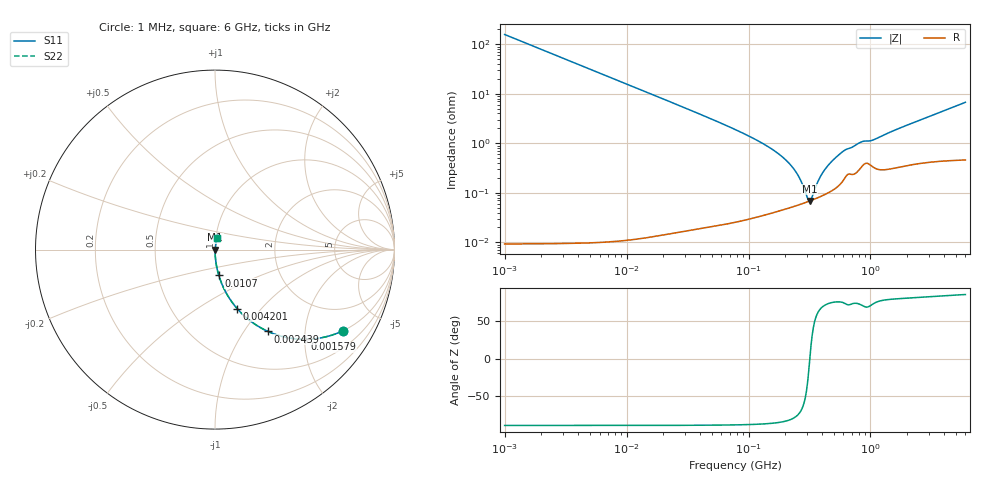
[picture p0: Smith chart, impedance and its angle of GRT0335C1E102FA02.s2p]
!Murata Part Number: GRT0335C1E102FA02
!These Parameters are Measured in Series Mode Connection
!Data Generated on Jun 19, 2026
!  o--ll--o
!Port1  Port2
!  o------o
!Operation Temp=25[degC], DC Bias Voltage=0[V]
!Freq. Start=1000[kHz] Stop=6[GHz] 401[Steps]
# Hz S RI R 50
!Freq.(Hz) S11(Real) S11(Imag) S21(Real) S21(Imag) S12(Real) S12(Imag) S22(Real) S22(Imag)
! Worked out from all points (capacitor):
!   401 points, 1 MHz to 6 GHz, reference 50 ohm
!   read as one part in series: C = 1.01 nF near 1.044 MHz
!   lowest |Z| = 68.5 mohm at 318.4 MHz (marker M1)
!   series resonance near 318.1 MHz, so ESL is about 250 pH
!   S11 on the Smith chart (normalised r, x): 1 MHz: 1.00, -3.15; 1.579 MHz: 1.00, -2.00; 2.439 MHz: 1.00, -1.29; 4.201 MHz: 1.00, -0.75; 10.7 MHz: 1.00, -0.29; 6 GHz: 1.01, +0.13
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1000000  0.7133 -0.4522  0.2867 0.4522  0.2867 0.4522  0.7133 -0.4522
1578894  0.4995 -0.5  0.5005 0.5  0.5005 0.5  0.4995 -0.5
2439274  0.2948 -0.4559  0.7052 0.4559  0.7052 0.4559  0.2948 -0.4559
4201409  0.1235 -0.3289  0.8765 0.3289  0.8765 0.3289  0.1235 -0.3289
4293785  0.1189 -0.3235  0.8811 0.3235  0.8811 0.3235  0.1189 -0.3235
1.0704e7  0.0213 -0.144  0.9787 0.144  0.9787 0.144  0.0213 -0.144
1.843659e7  0.00734 -0.0846  0.9927 0.0846  0.9927 0.0846  0.00734 -0.0846
7.745967e7  0.000615 -0.019  0.9994 0.019  0.9994 0.019  0.000615 -0.019
1.39348e8  0.000443 -0.00904  0.9996 0.00904  0.9996 0.00904  0.000443 -0.00904
2.016844e8  0.000491 -0.0046  0.9995 0.0046  0.9995 0.0046  0.000491 -0.0046
2.506837e8  0.000562 -0.00234  0.9994 0.00234  0.9994 0.00234  0.000562 -0.00234
2.734687e8  0.0006 -0.00148  0.9994 0.00148  0.9994 0.00148  0.0006 -0.00148
3.048839e8  0.000658 -0.000413  0.9993 0.000413  0.9993 0.000413  0.000658 -0.000413
3.184382e8  0.000685 1e-05  0.9993 -1e-05  0.9993 -1e-05  0.000685 1e-05
3.325952e8  0.000714 0.000433  0.9993 -0.000433  0.9993 -0.000433  0.000714 0.000433
3.708027e8  0.000798 0.00149  0.9992 -0.00149  0.9992 -0.00149  0.000798 0.00149
4.133993e8  0.000905 0.00258  0.9991 -0.00258  0.9991 -0.00258  0.000905 0.00258
5.60538e8  0.00149 0.0059  0.9985 -0.0059  0.9985 -0.0059  0.00149 0.0059
8.291285e8  0.00324 0.00994  0.9968 -0.00994  0.9968 -0.00994  0.00324 0.00994
1.053225e9  0.0034 0.0111  0.9966 -0.0111  0.9966 -0.0111  0.0034 0.0111
1.428092e9  0.00326 0.0162  0.9967 -0.0162  0.9967 -0.0162  0.00326 0.0162
6e9  0.00901 0.0663  0.991 -0.0663  0.991 -0.0663  0.00901 0.0663
